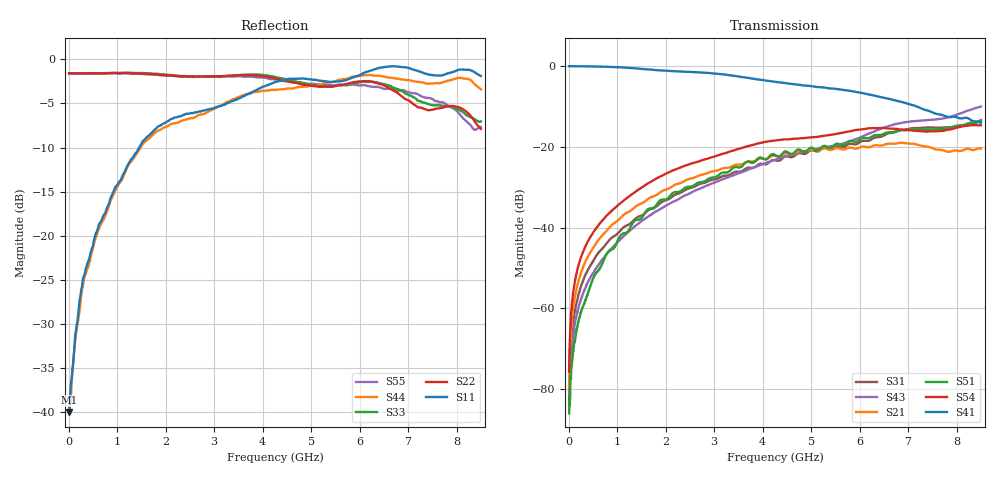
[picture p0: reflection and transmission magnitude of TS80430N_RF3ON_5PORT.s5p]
!Created with skrf (http://scikit-rf.org).
# GHz S RI R 50.0
!freq ReS11 ImS11 ReS12 ImS12 ReS13 ImS13
! ReS14 ImS14 ReS15 ImS15
! ReS21 ImS21 ReS22 ImS22 ReS23 ImS23
! ReS24 ImS24 ReS25 ImS25
! ReS31 ImS31 ReS32 ImS32 ReS33 ImS33
! ReS34 ImS34 ReS35 ImS35
! ReS41 ImS41 ReS42 ImS42 ReS43 ImS43
! ReS44 ImS44 ReS45 ImS45
! ReS51 ImS51 ReS52 ImS52 ReS53 ImS53
! ReS54 ImS54 ReS55 ImS55
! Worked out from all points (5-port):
!   1601 points, 10 MHz to 8.5 GHz, reference 50 ohm
!   strongest paths, dB at 10 MHz, 2.132 GHz, 4.255 GHz, 6.378 GHz, 8.5 GHz:
!     S41: -0.1, -1.3, -4.0, -7.6, -14.2
!     S54: -75.5, -26.0, -18.5, -15.4, -14.7
!     S51: -85.9, -31.6, -22.1, -17.1, -13.7
!     S21: -79.5, -29.8, -22.3, -19.7, -20.5
!     S43: -81.3, -33.8, -23.2, -15.9, -10.1
!     S31: -84.0, -32.4, -23.3, -17.7, -13.4
!   lowest |S11| = -40.0 dB at 15.31 MHz (marker M1), VSWR 1.02, Z = 50.9 - j0.353 ohm
!   |S11| at or under -10 dB: start of sweep to 1.453 GHz
